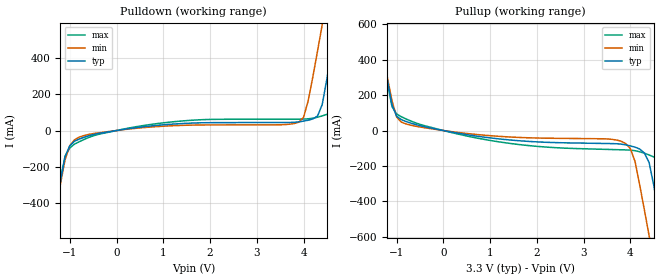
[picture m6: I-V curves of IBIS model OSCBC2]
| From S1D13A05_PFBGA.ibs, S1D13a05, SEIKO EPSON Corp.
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[Model]   OSCBC2
Model_type Output
Polarity Non-Inverting
C_comp   5p   4p   6p
[Temperature Range] 50   100   0
[Voltage Range]   3.3   3.0   3.6
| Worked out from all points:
|   slope of the pulldown table from 0 to 0.495 V, typ, clamps not added: 27.1 ohm
|   slope of the pullup table from 0 to 0.495 V, typ, clamps not added: 21.5 ohm
[Pullup]
-3.3V     3.65A      3.36A      4A
-1.4V     601mA      588.4mA    617.5mA
-1.1V     144.8mA    167.9mA    134.5mA
-1V       80.13mA    75.7mA     93.28mA
-800mV    50.98mA    37.1mA     65.36mA
1.3V      -50.18mA   -34.56mA   -68.1mA
3.9V      -80.76mA   -73.49mA   -109.4mA
4.1V      -93.87mA   -174.7mA   -113.8mA
4.4V      -179.3mA   -591.9mA   -137.6mA
4.7V      -621.1mA   -1.026A    -207.5mA
5V        -1.101A    -1.461A    -663.3mA
6.6V      -3.674A    -3.796A    -3.537A
[Pulldown]
-3.3V     -3.648A    -3.346A    -4.034A
-1.4V     -593mA     -579.2mA   -617.6mA
-1.1V     -141.9mA   -158.9mA   -140.3mA
-1V       -84.28mA   -82.28mA   -95.46mA
-800mV    -46.77mA   -36.14mA   -61.64mA
1.2V      35.15mA    26.31mA    47.76mA
3.9V      47.68mA    45.86mA    62.66mA
4.1V      56.62mA    163.3mA    64.29mA
4.4V      142.4mA    580.8mA    80.25mA
4.7V      595.8mA    1.015A     139.3mA
5V        1.075A     1.451A     618.1mA
6.6V      3.639A     3.781A     3.466A
[Ramp]
R_load=50
dV/dt_r   1.327E+0/8.088E-10   1.029E+0/7.871E-10   1.595E+0/8.438E-10
dV/dt_f   1.145E+0/7.864E-10   8.802E-1/9.601E-10   1.437E+0/7.065E-10
